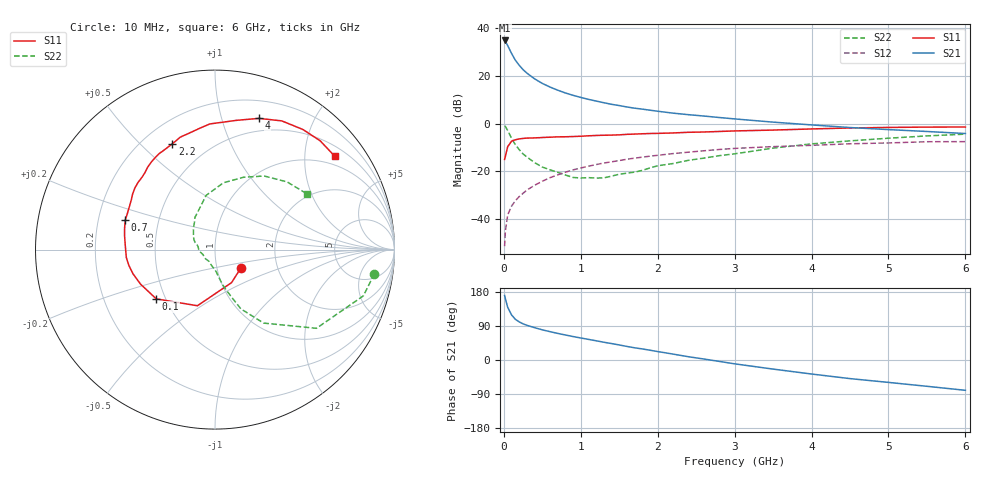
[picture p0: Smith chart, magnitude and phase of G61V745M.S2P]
! SIEMENS Small Signal Semiconductors
! BFG193
! Si NPN RF Bipolar Junction Transistor in SOT223
! VCE = 1.75 V  IC = 45 mA
! Common Emitter S-Parameters:  August  1996
# GHz  S  MA  R  50
!  f  S11  S21  S12  S22
! GHz  MAG  ANG  MAG  ANG  MAG  ANG  MAG  ANG
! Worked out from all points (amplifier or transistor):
!   36 points, 10 MHz to 6 GHz, reference 50 ohm
!   highest |S21| = 34.8 dB at 10 MHz (marker M1)
!   |S21| within 3 dB of that: start of sweep to 63.18 MHz
!   unconditionally stable (mu >= 1): 378.4 MHz to 2.639 GHz
!   at 250 MHz: K = 0.93, MSG = 25.9 dB, |S12| = -29.2 dB
!   at 1.4 GHz: K = 1.06, MAG = 10.5 dB, |S12| = -16.0 dB
!   at 6 GHz: K = 0.94, MSG = 1.7 dB, |S12| = -7.6 dB
!   S11 on the Smith chart (normalised r, x): 10 MHz: 1.30, -0.28; 100 MHz: 0.45, -0.30; 700 MHz: 0.32, +0.15; 2.2 GHz: 0.32, +0.63; 4 GHz: 0.37, +1.32; 6 GHz: 0.75, +2.73
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0.01  0.1771 -35.6  55.04 170.2  0.0027 87.6  0.8983 -8.6
0.02  0.206 -63.5  52.55 161.6  0.0056 76.7  0.866 -17.3
0.05  0.3278 -107.4  43.07 139.1  0.0122 67.4  0.7154 -37.8
0.1  0.4271 -140.0  29.45 119.1  0.0186 63.3  0.491 -56.5
0.15  0.457 -155.0  21.21 107.3  0.0242 63.0  0.3606 -66.4
0.2  0.4766 -163.6  16.6 100.6  0.0295 64.6  0.2845 -70.5
0.25  0.4881 -169.7  13.46 95.4  0.0346 65.5  0.2306 -74.8
0.3  0.496 -174.9  11.38 91.5  0.0405 66.7  0.1995 -77.8
0.4  0.5001 177.7  8.636 85.3  0.0509 66.8  0.1519 -82.7
0.5  0.5099 171.2  6.931 79.6  0.0619 66.3  0.1227 -87.1
0.6  0.5177 166.6  5.817 74.8  0.0735 65.2  0.1073 -92.0
0.7  0.5264 161.7  5.003 70.2  0.0841 64.1  0.095 -99.4
0.9  0.5346 152.9  3.904 61.9  0.107 60.4  0.0743 -115.1
1.1  0.5536 146.0  3.213 54.4  0.1278 56.6  0.0736 -135.7
1.6  0.5935 129.1  2.224 35.8  0.1788 45.3  0.0914 178.4
2.2  0.6354 112.0  1.652 15.6  0.2349 31.1  0.1453 145.7
2.8  0.6828 96.8  1.338 -3.7  0.2863 16.8  0.2123 121.6
3.5  0.7299 80.6  1.071 -24.0  0.3287 -0.9  0.3056 99.4
4  0.7709 71.5  0.936 -37.0  0.3495 -10.7  0.3754 82.8
4.5  0.8078 62.6  0.825 -49.1  0.377 -20.8  0.4337 68.4
5.5  0.8432 45.9  0.682 -69.4  0.416 -43.8  0.551 43.2
6  0.846 37.9  0.618 -80.0  0.4182 -56.9  0.6004 31.0
